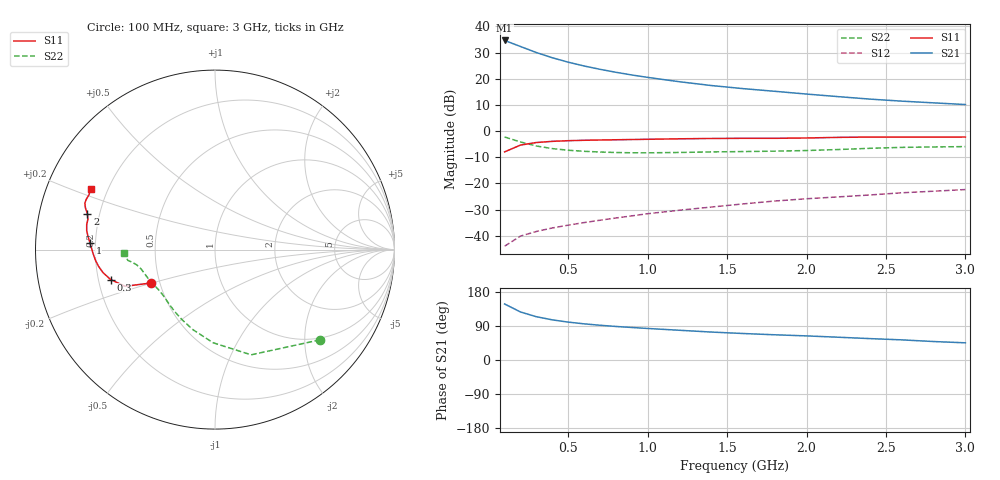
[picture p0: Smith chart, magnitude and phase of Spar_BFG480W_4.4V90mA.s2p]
! Filename: 4_490BFG480.001
! Title: BFG480W
! Bias: Vce=4.4V; Ic=90mA
! Company: NXP Semiconductors NL
! User: Quality&Reliability T&D
! Measure time: 10 Nov 1999 / 12:06:50
#  MHz  S  MA  R 50
! Freq  S11  S21  S12  S22  :
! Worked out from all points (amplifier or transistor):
!   20 points, 100 MHz to 3 GHz, reference 50 ohm
!   highest |S21| = 34.6 dB at 100 MHz (marker M1)
!   |S21| within 3 dB of that: start of sweep to 229.9 MHz
!   unconditionally stable (mu >= 1): 764.2 MHz to end of sweep
!   at 400 MHz: K = 0.78, MSG = 32.5 dB, |S12| = -37.0 dB
!   at 1.2 GHz: K = 1.07, MAG = 22.9 dB, |S12| = -30.2 dB
!   at 3 GHz: K = 1.04, MAG = 14.9 dB, |S12| = -22.3 dB
!   S11 on the Smith chart (normalised r, x): 100 MHz: 0.45, -0.20; 300 MHz: 0.25, -0.13; 1 GHz: 0.18, +0.03; 2 GHz: 0.15, +0.14; 3 GHz: 0.14, +0.23
100  0.4012 -152.4  53.91 147.8  0.006334 68.6  0.7716 -40.7
200  0.5411 -157.8  41.32 126.7  0.009876 59.9  0.6199 -71.0
300  0.6051 -164.0  31.68 114.2  0.01209 58.2  0.5191 -91.2
400  0.6372 -168.4  25.19 106.0  0.0141 59.5  0.4631 -105.3
500  0.6558 -171.9  20.76 100.0  0.01596 61.8  0.4308 -115.5
600  0.6677 -174.7  17.54 95.4  0.01787 63.5  0.4113 -123.2
700  0.6762 -177.1  15.16 91.7  0.01982 65.8  0.3984 -129.2
800  0.683 -179.2  13.3 88.5  0.02186 67.7  0.3899 -134.3
900  0.6902 178.8  11.82 85.8  0.02401 69.5  0.3854 -138.6
1000  0.6978 177.0  10.63 83.2  0.02639 70.6  0.3845 -142.5
1200  0.7124 173.9  8.773 78.5  0.03078 72.5  0.3906 -148.8
1400  0.7229 171.5  7.429 73.8  0.03538 73.6  0.4004 -153.5
1600  0.728 169.1  6.48 69.9  0.04061 74.5  0.4066 -157.1
1800  0.7282 166.5  5.76 66.5  0.04614 75.2  0.4138 -160.8
2000  0.7388 164.2  5.1 63.6  0.05101 75.8  0.4253 -165.2
2200  0.7588 162.1  4.553 60.1  0.05533 75.9  0.4444 -169.0
2400  0.7697 160.4  4.083 56.4  0.06026 75.4  0.4691 -171.5
2600  0.77 158.7  3.733 53.1  0.06631 74.8  0.4886 -172.9
2800  0.7656 156.5  3.463 48.7  0.07106 73.4  0.498 -174.8
3000  0.7705 153.8  3.216 45.3  0.07645 72.7  0.5056 -177.7
